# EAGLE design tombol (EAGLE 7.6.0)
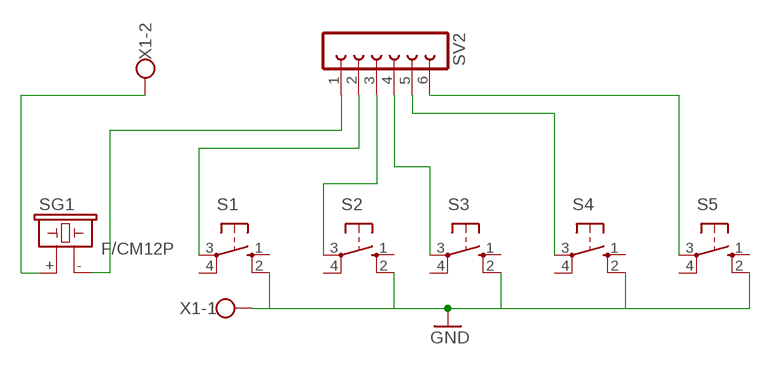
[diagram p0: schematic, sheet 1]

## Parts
S1  40-XX  [B3F-40XX]
S2  40-XX  [B3F-40XX]
S3  40-XX  [B3F-40XX]
S4  40-XX  [B3F-40XX]
S5  40-XX  [B3F-40XX]
SG1  F/CM12P  [F/CM12P]
SV2  FE06-1  [FE06]
X1  W237-102  [W237-102]

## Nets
GND: S1.2(S1) S2.2(S1) S3.2(S1) S4.2(S1) S5.2(S1) X1.1
N$1: S5.3(P) SV2.6
N$2: S4.3(P) SV2.5
N$3: S3.3(P) SV2.4
N$4: S2.3(P) SV2.3
N$5: S1.3(P) SV2.2
N$6: SG1.+ X1.2
N$7: SG1.- SV2.1
Unconnected: S1.1(S) S1.4(P1) S2.1(S) S2.4(P1) S3.1(S) S3.4(P1) S4.1(S) S4.4(P1) S5.1(S) S5.4(P1)

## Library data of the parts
S1-S5 = switch-omron:40-XX: OMRON SWITCH; MF: OMRON COMPONENTS USA; MPN: B3F-4000; OC_FARNELL: 176434; OC_NEWARK: 36K3105
SG1 = buzzer:F/CM12P: BUZZER; OC_FARNELL: unknown; OC_NEWARK: unknown
SV2 = con-lsta:FE06-1: FEMALE HEADER; OC_FARNELL: unknown; OC_NEWARK: unknown
X1 = con-wago-500:W237-102: WAGO SCREW CLAMP; MPN: 237-102; OC_FARNELL: unknown; OC_NEWARK: 70K9898

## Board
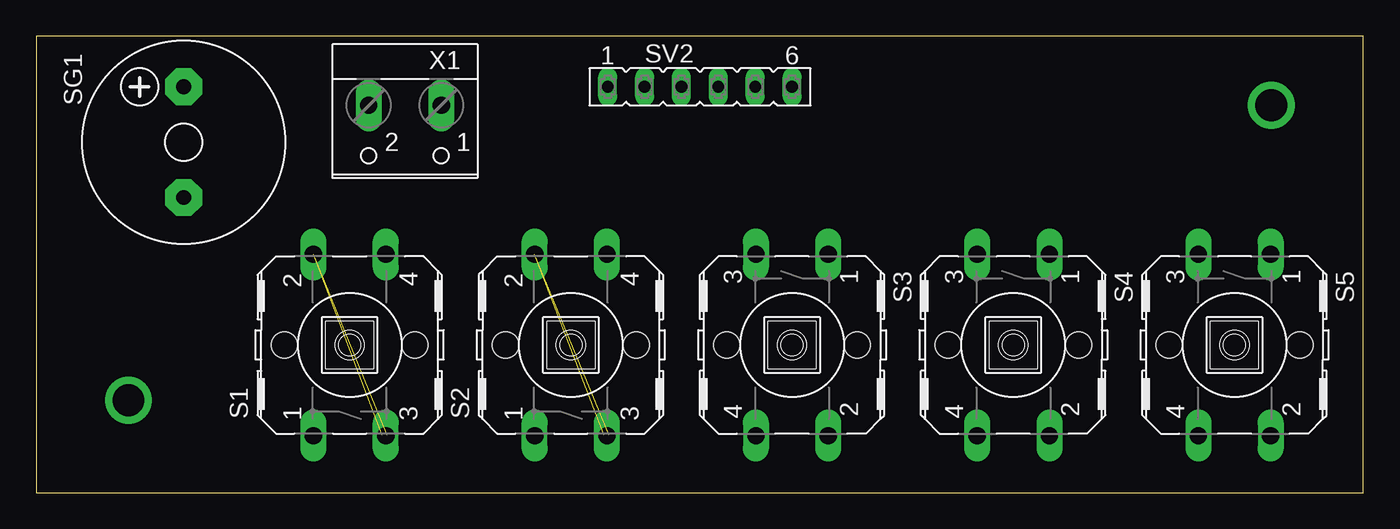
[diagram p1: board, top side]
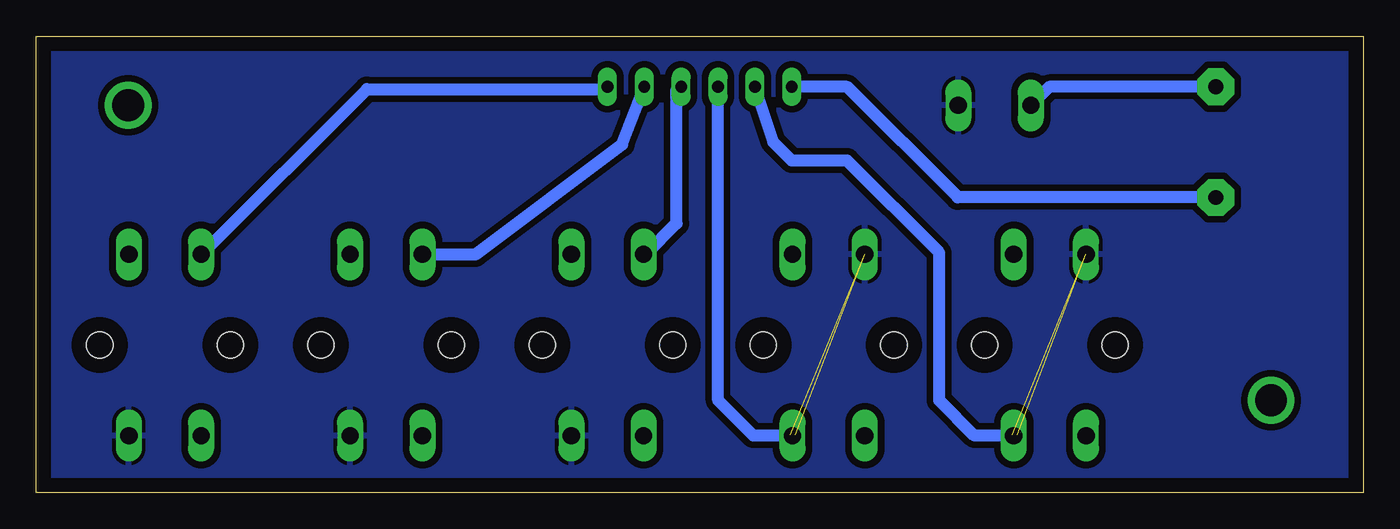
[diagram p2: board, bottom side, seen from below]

Size 91.42 x 31.42 mm. Coordinates in mm from the lower left corner, seen from the top.
Outline: 0,0 91.42,0 91.42,31.42 0,31.42 0,0
Copper layers (1*16): Top 0.035mm / dielectric 1.5mm / Bottom 0.035mm
Design rules "default *": minimum track width 10mil, minimum drill 24mil, track to track 18mil, track to pad 18mil, pad to pad 18mil, via to via 18mil, smd to smd 8mil, copper to edge 40mil, drill to drill 8mil, minimum pad ring 10mil, minimum via ring 8mil, stop-mask expansion 4mil, vias tented up to drill 0mil, thermal gap 10mil

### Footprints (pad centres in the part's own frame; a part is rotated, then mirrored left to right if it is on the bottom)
B3F-40XX = drill 1.194 long: 1 -6.248,2.489; 2 6.248,2.489; 3 -6.248,-2.489; 4 6.248,-2.489 | hole 1.803: 0,-4.496; 0,4.496
F/CM12P = drill 1.016 pad 2.54 octagon: + 3.81,0; - -3.81,0
FE06 = drill 0.813 long: 1 -6.35,0; 2 -3.81,0; 3 -1.27,0; 4 1.27,0; 5 3.81,0; 6 6.35,0
W237-102 = drill 1.194 long: 1 -2.5,-1.27; 2 2.5,-1.27

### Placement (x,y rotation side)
S1  21.59,10.16 90 top
S2  36.83,10.16 90 top
S3  52.07,10.16 270 top
S4  67.31,10.16 270 top
S5  82.55,10.16 270 top
SG1  10.16,24.13 90 top
SV2  45.72,27.94 0 top
X1  25.4,25.4 180 top

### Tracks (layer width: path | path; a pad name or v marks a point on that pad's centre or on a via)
GND  (4 unrouted)
  pour Bottom: 0,31.75 91.44,31.75 91.44,0 0,0
N$1
  Bottom 0.254: 52.27,27.79 SV2.6 | 80.01,16.41 S5.3
  Bottom 0.813: 52.27,27.79 68.63,27.79 80.01,16.41
N$2
  Bottom 0.813: S4.3 61.16,16.41 51.05,23.98 SV2.5
N$3
  Bottom 0.254: 47.3,27.79 SV2.4 | 49.43,16.41 S3.3
  Bottom 0.813: 47.3,27.79 47.3,18.54 49.43,16.41
N$4
  Bottom 0.813: S2.3 42.01,3.91 44.45,6.35 SV2.3
N$5
  Bottom 0.813: S1.3 26.77,3.91 29.21,6.35 29.21,16.51 35.56,22.86 39.37,22.86 40.64,24.13 SV2.2
N$6
  Bottom 0.813: SG1.+ 21.63,27.94 X1.2
N$7
  Bottom 0.813: SG1.- 27.94,20.32 35.56,27.94 SV2.1
N$8  (via drill 2.2 pad 1.68)
  other vias: 85.09,26.67
N$9  (via drill 2.2 pad 1.68)
  other vias: 6.35,6.35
